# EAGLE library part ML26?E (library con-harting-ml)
HARTING
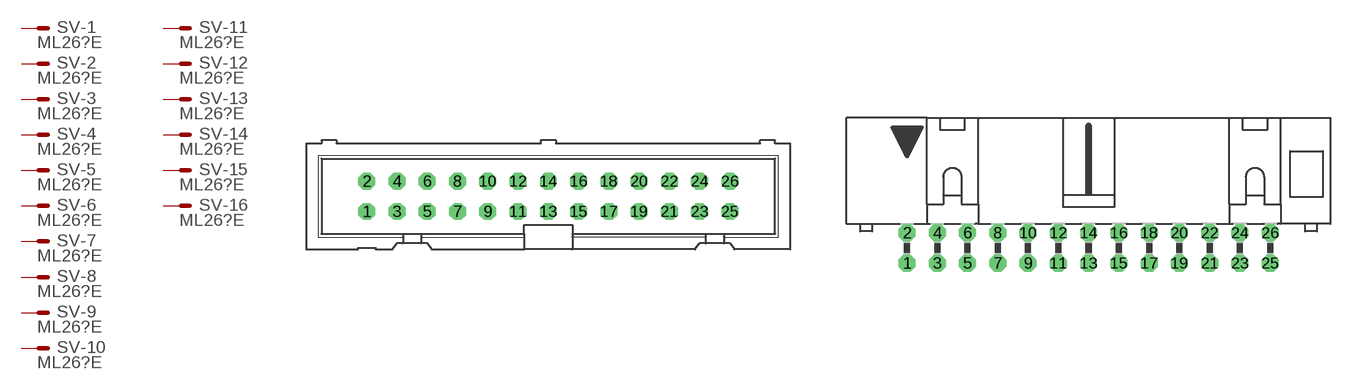
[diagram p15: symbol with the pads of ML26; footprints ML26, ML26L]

Designator prefix SV; gates -1=M -2=M -3=M -4=M -5=M -6=M -7=M -8=M -9=M -10=M -11=M -12=M -13=M -14=M -15=M -16=M -17=M -18=M -19=M -20=M -21=M -22=M -23=M -24=M -25=M -26=M

## ML26E (OC_FARNELL: unknown; OC_NEWARK: unknown)  [ML26]
1  -1:S  pas
2  -2:S  pas
3  -3:S  pas
4  -4:S  pas
5  -5:S  pas
6  -6:S  pas
7  -7:S  pas
8  -8:S  pas
9  -9:S  pas
10  -10:S  pas
11  -11:S  pas
12  -12:S  pas
13  -13:S  pas
14  -14:S  pas
15  -15:S  pas
16  -16:S  pas
17  -17:S  pas
18  -18:S  pas
19  -19:S  pas
20  -20:S  pas
21  -21:S  pas
22  -22:S  pas
23  -23:S  pas
24  -24:S  pas
25  -25:S  pas
26  -26:S  pas

## ML26LE (OC_FARNELL: unknown; OC_NEWARK: unknown)  [ML26L]
Pads as for ML26

## ML263ME (OC_FARNELL: unknown; OC_NEWARK: unknown)  [3M_26]
Pads as for ML26

## ML263MLE (OC_FARNELL: unknown; OC_NEWARK: unknown)  [3M_26L]
Pads as for ML26

## Footprint ML26 (pad centres in mm)
HARTING
drill 0.914 octagon: 1 -15.24,-1.27; 2 -15.24,1.27; 3 -12.7,-1.27; 4 -12.7,1.27; 5 -10.16,-1.27; 6 -10.16,1.27; 7 -7.62,-1.27; 8 -7.62,1.27; 9 -5.08,-1.27; 10 -5.08,1.27; 11 -2.54,-1.27; 12 -2.54,1.27; 13 0,-1.27; 14 0,1.27; 15 2.54,-1.27; 16 2.54,1.27; 17 5.08,-1.27; 18 5.08,1.27; 19 7.62,-1.27; 20 7.62,1.27; 21 10.16,-1.27; 22 10.16,1.27; 23 12.7,-1.27; 24 12.7,1.27; 25 15.24,-1.27; 26 15.24,1.27

## Footprint ML26L (pad centres in mm)
HARTING
drill 0.914 octagon: 1 -15.24,-1.27; 2 -15.24,1.27; 3 -12.7,-1.27; 4 -12.7,1.27; 5 -10.16,-1.27; 6 -10.16,1.27; 7 -7.62,-1.27; 8 -7.62,1.27; 9 -5.08,-1.27; 10 -5.08,1.27; 11 -2.54,-1.27; 12 -2.54,1.27; 13 0,-1.27; 14 0,1.27; 15 2.54,-1.27; 16 2.54,1.27; 17 5.08,-1.27; 18 5.08,1.27; 19 7.62,-1.27; 20 7.62,1.27; 21 10.16,-1.27; 22 10.16,1.27; 23 12.7,-1.27; 24 12.7,1.27; 25 15.24,-1.27; 26 15.24,1.27

## Footprint 3M_26 (pad centres in mm)
3M
drill 0.813 square: 1 -15.24,-1.27; 2 -15.24,1.27; 3 -12.7,-1.27; 4 -12.7,1.27; 5 -10.16,-1.27; 6 -10.16,1.27; 7 -7.62,-1.27; 8 -7.62,1.27; 9 -5.08,-1.27; 10 -5.08,1.27; 11 -2.54,-1.27; 12 -2.54,1.27; 13 0,-1.27; 14 0,1.27; 15 2.54,-1.27; 16 2.54,1.27; 17 5.08,-1.27; 18 5.08,1.27; 19 7.62,-1.27; 20 7.62,1.27; 21 10.16,-1.27; 22 10.16,1.27; 23 12.7,-1.27; 24 12.7,1.27; 25 15.24,-1.27; 26 15.24,1.27

## Footprint 3M_26L (pad centres in mm)
3M
drill 0.813 square: 1 -15.24,-5.08; 2 -15.24,-2.54; 3 -12.7,-5.08; 4 -12.7,-2.54; 5 -10.16,-5.08; 6 -10.16,-2.54; 7 -7.62,-5.08; 8 -7.62,-2.54; 9 -5.08,-5.08; 10 -5.08,-2.54; 11 -2.54,-5.08; 12 -2.54,-2.54; 13 0,-5.08; 14 0,-2.54; 15 2.54,-5.08; 16 2.54,-2.54; 17 5.08,-5.08; 18 5.08,-2.54; 19 7.62,-5.08; 20 7.62,-2.54; 21 10.16,-5.08; 22 10.16,-2.54; 23 12.7,-5.08; 24 12.7,-2.54; 25 15.24,-5.08; 26 15.24,-2.54
hole 2.54 at -21.158,-3.277
hole 2.54 at 21.158,-3.277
